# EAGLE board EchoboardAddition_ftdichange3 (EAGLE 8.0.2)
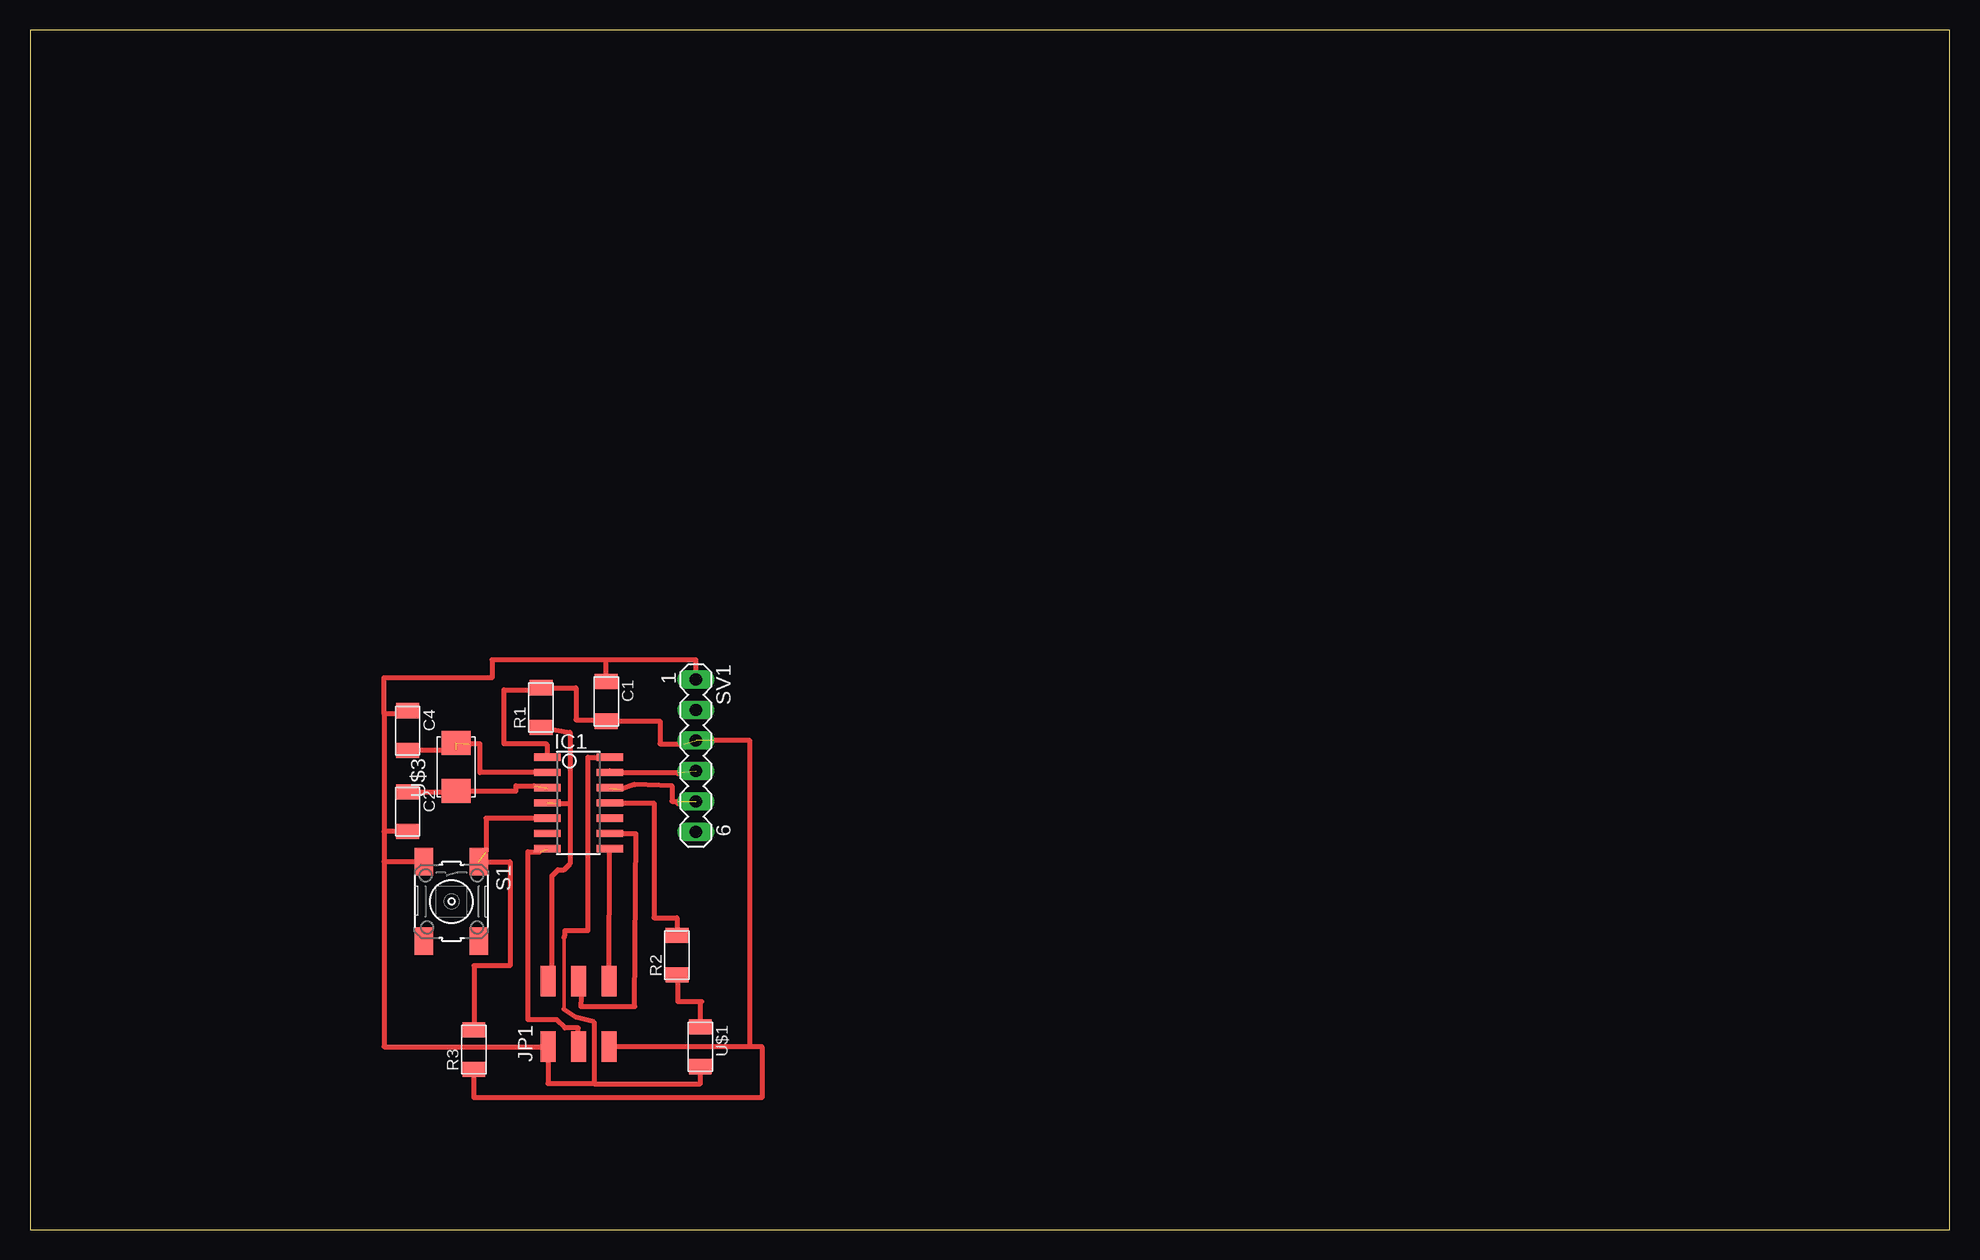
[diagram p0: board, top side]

Size 160 x 100 mm. Coordinates in mm from the lower left corner, seen from the top.
Outline: 0,0 160,0 160,100 0,100 0,0
Copper layers (1*16): Top 0.035mm / dielectric 1.5mm / Bottom 0.035mm
Design rules "default *": minimum track width 10mil, minimum drill 24mil, track to track 0.4mm, track to pad 0.4mm, pad to pad 0.4mm, via to via 0.4mm, smd to smd 0.4mm, copper to edge 40mil, drill to drill 8mil, minimum pad ring 10mil, minimum via ring 8mil, stop-mask expansion 4mil, vias tented up to drill 0mil, thermal gap 10mil

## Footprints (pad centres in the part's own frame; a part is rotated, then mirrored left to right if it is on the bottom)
C1206FAB = smd 1.27 x 1.905: 1 -1.651,0; 2 1.651,0
SOIC14 = smd 0.61 x 2.21: 1 -3.81,-2.603; 2 -2.54,-2.603; 3 -1.27,-2.603; 4 0,-2.603; 5 1.27,-2.603; 6 2.54,-2.603; 7 3.81,-2.603; 8 3.81,2.603; 9 2.54,2.603; 10 1.27,2.603; 11 0,2.603; 12 -1.27,2.603; 13 -2.54,2.603; 14 -3.81,2.603
2X03SMD = smd 2.54 x 1.27: 1 -2.54,2.54; 2 2.92,2.54; 3 -2.54,0; 4 2.92,0; 5 -2.54,-2.54; 6 2.92,-2.54
R1206FAB = smd 1.27 x 1.905: 1 -1.651,0; 2 1.651,0
6MM_SWITCH = smd 2.286 x 1.524: 1 -3.302,2.286; 2 3.302,2.286; 3 -3.302,-2.286; 4 3.302,-2.286
MA06-1 = drill 1.016 long: 1 -6.35,0; 2 -3.81,0; 3 -1.27,0; 4 1.27,0; 5 3.81,0; 6 6.35,0
LED1206FAB = smd 1.27 x 1.905: 1 -1.651,0; 2 1.651,0
2-SMD-5X3MM = smd 2 x 2.4: P$1 -2,0; P$2 2,0

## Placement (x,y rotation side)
C1  1microF  [C1206FAB]  48.03,44.03 270 top
C2  [C1206FAB]  31.48,34.83 270 top
C4  [C1206FAB]  31.48,41.59 270 top
IC1  ATTINY44-SSU  [SOIC14]  45.72,35.56 270 top
JP1  [2X03SMD]  45.72,17.78 90 top
R1  10k  [R1206FAB]  42.59,43.51 90 top
R2  [R1206FAB]  53.93,22.87 90 top
R3  [R1206FAB]  37,15 90 top
S1  [6MM_SWITCH]  35.13,27.35 270 top
SV1  [MA06-1]  55.5,39.5 270 top
U$1  LEDFAB1206  [LED1206FAB]  55.88,15.24 270 top
U$3  CRYSTAL  [2-SMD-5X3MM]  35.52,38.55 90 top

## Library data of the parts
C1 C2 C4 IC1 JP1 R1-R3 S1 U$1 U$3 = fab
SV1 = con-lstb; OC_FARNELL: unknown; OC_NEWARK: unknown

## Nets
GND: C1.1 C2.2 C4.1 IC1.14 JP1.1 S1.3 SV1.1 U$1.2
LED_PA2: IC1.11 R2.2
MISO_PA5: IC1.8 JP1.6
MOSI_PA6: IC1.7 JP1.3
N$3: R2.1 U$1.1
RST: IC1.4 JP1.2 R1.1
RX_PA1: IC1.12 SV1.5
SCK_PA4: IC1.9 JP1.4
SW_B2: IC1.5 R3.2 S1.1
TX_PA0: IC1.13 SV1.4
U3_PB0: C4.2 IC1.2 U$3.P$2
U3_PB1: C2.1 IC1.3 U$3.P$1
VCC: C1.2 IC1.1 JP1.5 R1.2 R3.1 SV1.3

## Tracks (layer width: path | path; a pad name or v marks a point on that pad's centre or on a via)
GND
  Top 0.305: 44.5,24.34 44.5,18.36
  Top 0.406: 47,12.16 55.88,12.16 U$1.2 55.88,13.5 56.5,13.5 | 47,12.16 43.18,12.16 JP1.1 29.5,15.24 29.5,30.65 | 48.32,39.5 IC1.14 46.5,39.37 46.5,24.94 44.6,24.94 44.5,24.34 | 47,12.16 47,17.3 45.5,17.7 44.5,18.36 | 48,47.5 38.5,47.5 38.5,46 29.5,46 29.5,43 | 48,47.5 55.5,47.5 SV1.1 | 29.5,33.18 29.5,30.65 | 29.5,43 29.5,33.18 | S1.3 29.5,30.65 | C2.2 29.5,33.18 | C4.1 31,43.24 31,43 29.5,43 | C1.1 48,45.68 48,47.5
LED_PA2
  Top 0.406: IC1.11 52,35.56 52,26 53.93,26 R2.2
MISO_PA5
  Top 0.406: JP1.6 IC1.8
MOSI_PA6  (1 unrouted)
  Top 0.406: 45.5,15.24 JP1.3 45.7,15.24 45.7,16.8 44.6,16.8 43.9,17.5 41.5,17.5 41.5,31.5 42.5,31.5
N$3
  Top 0.406: U$1.1 55.88,19 56,19 54,19 54,21.22 R2.1
RST  (1 unrouted)
  Top 0.406: 43,20 43,20.52 JP1.2 43.5,21.02 43.5,29.5 44,30 44.5,30 45,30.5 45,35.5 | 45,35.5 44,35.5 | R1.1 45,41.45 45,35.5
RX_PA1  (2 unrouted)
  Top 0.406: 49.2,36.7 50.4,37.1 53.5,37 53.5,35.69 54,35.69 54,35.5
SCK_PA4
  Top 0.406: IC1.9 49,33 50.5,33 50.4,18.6 45.9,18.6 46,20.7 JP1.4
SW_B2  (1 unrouted)
  Top 0.406: R3.2 37,22 40,22 40,30.65 S1.1 | IC1.5 38,34.29 38,31.5
TX_PA0  (1 unrouted)
  Top 0.406: 48.32,38.23 IC1.13 54,38.1 54,38
U3_PB0  (2 unrouted)
  Top 0.406: IC1.2 37.5,38.1 37.5,40.5 36.6,40.5 36.6,40.3 | C4.2 35.5,39.94 35.5,40
U3_PB1  (1 unrouted)
  Top 0.406: C2.1 35.52,36.48 U$3.P$1 40.5,36.55 40.5,37 42,37
VCC  (2 unrouted)
  Top 0.406: 60,15.24 61,15.24 61,11 37,11 R3.1 | 60,15.24 JP1.5 | IC1.1 43.12,40.38 43,40.5 39.5,40.5 39.5,45 42.59,45 R1.2 45.5,45.16 45.5,42.5 48.03,42.5 C1.2 52.5,42.38 52.5,40.5 54.5,40.5 | 60,15.24 60,40.77 57,40.77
